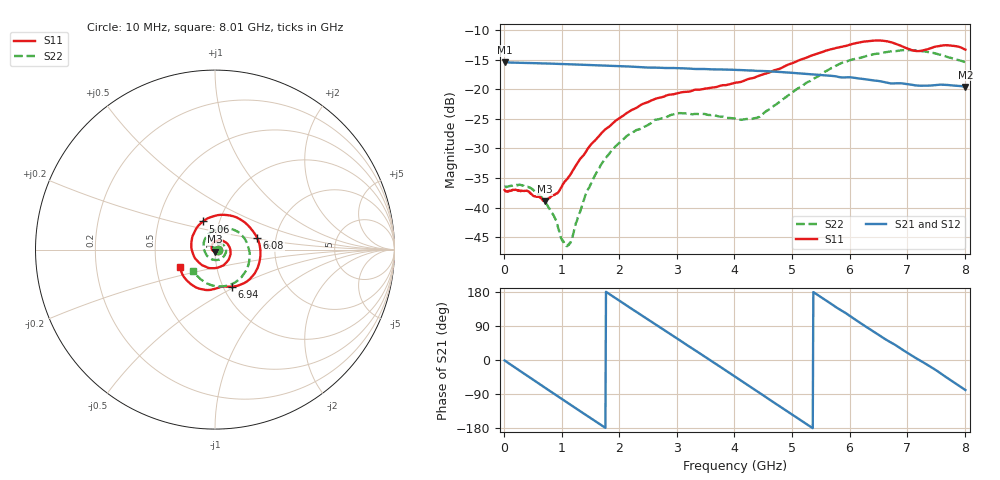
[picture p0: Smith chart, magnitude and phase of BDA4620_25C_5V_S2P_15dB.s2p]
!Agilent Technologies,E5071B,MY42404982,A.09.10
!Date: Wed May 06 09:01:22 2026
!Data & Calibration Information:
!Freq	S11:SOLT2(ON)	S21:SOLT2(ON)	S12:SOLT2(ON)	S22:SOLT2(ON)
# Hz S RI R 50
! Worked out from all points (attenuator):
!   801 points, 10 MHz to 8.01 GHz, reference 50 ohm
!   highest |S21| = -15.42 dB at 10 MHz (marker M1); lowest = -19.6 dB at 8.01 GHz (marker M2)
!   lowest |S11| = -38.9 dB at 710 MHz (marker M3), VSWR 1.02, Z = 49.8 - j1.11 ohm
!   |S11| at or under -10 dB: start of sweep to end of sweep
!   |S22| runs from -46.5 to -13.4 dB; largest |S21 - S12| = 0.00078
!   S11 on the Smith chart (normalised r, x): 10 MHz: 1.03, -0.00; 5.06 GHz: 0.84, +0.27; 6.08 GHz: 1.59, +0.22; 6.94 GHz: 1.10, -0.48; 8.01 GHz: 0.66, -0.13
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1e7  0.0141 -0.000935  0.1693 -0.00361  0.1695 -0.00372  0.0151 -0.000645
4.4e8  0.00864 -0.0104  0.117 -0.1187  0.1171 -0.1189  0.0132 -0.0066
7.1e8  -0.00204 -0.0112  0.0485 -0.158  0.0484 -0.1583  0.00703 -0.00879
1.09e9  -0.0173 0.00112  -0.06 -0.1517  -0.06 -0.1517  -0.00383 -0.00278
1.17e9  -0.0187 0.0064  -0.0804 -0.1412  -0.0806 -0.1413  -0.00532 -0.000128
1.35e9  -0.0191 0.0187  -0.1196 -0.1082  -0.1198 -0.1083  -0.00728 0.0071
1.59e9  -0.0108 0.0358  -0.1519 -0.0493  -0.1521 -0.0493  -0.00537 0.0184
1.89e9  0.0129 0.0501  -0.1541 0.0332  -0.1543 0.0334  0.00582 0.0306
2.68e9  0.0844 0.00418  0.00243 0.1521  0.00261 0.1524  0.0526 0.0182
3.4e9  0.0373 -0.0919  0.1418 0.0444  0.142 0.0443  0.0456 -0.0416
4.01e9  -0.0774 -0.0826  0.1051 -0.1011  0.1052 -0.1014  -0.021 -0.0527
4.42e9  -0.1298 -0.00126  0.0123 -0.1426  0.012 -0.1428  -0.0573 -0.0103
5.06e9  -0.0666 0.1568  -0.1186 -0.0691  -0.119 -0.0691  -0.0267 0.0946
5.35e9  0.0201 0.1926  -0.1338 -0.00265  -0.1338 -0.00265  0.0283 0.1169
5.68e9  0.1331 0.1727  -0.1103 0.0687  -0.1104 0.0689  0.1008 0.1118
6.08e9  0.2348 0.0658  -0.0392 0.1188  -0.0392 0.1191  0.1749 0.0436
6.39e9  0.2493 -0.0632  0.0259 0.1164  0.0259 0.1165  0.1936 -0.0329
6.68e9  0.1845 -0.1726  0.0733 0.0856  0.0737 0.0858  0.1769 -0.1087
6.94e9  0.0944 -0.2068  0.1013 0.0471  0.1015 0.0471  0.134 -0.1668
7.2e9  0.0347 -0.2076  0.1073 0.00143  0.1076 0.00145  0.0658 -0.2015
7.58e9  -0.0773 -0.2201  0.0893 -0.0632  0.0896 -0.0632  -0.0376 -0.1919
8.01e9  -0.194 -0.0955  0.0196 -0.103  0.0196 -0.1033  -0.1208 -0.1175
